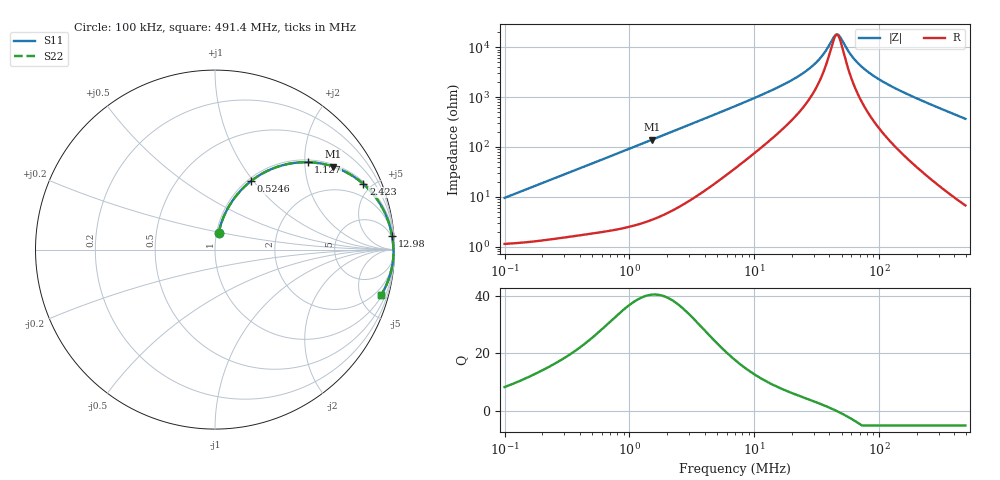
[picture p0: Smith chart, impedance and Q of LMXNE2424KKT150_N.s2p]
! LMXNE2424KKT150_N  S-PARAMETER MODEL  ( General Type )
! Model Generated by TAIYO YUDEN Corporation (http://www.ty-top.com)
! Version 1.0
! TAIYO YUDEN Control No. 191023NI43SB-FBB
! Copyright(c) 2019 TAIYO YUDEN CO.,LTD. All Rights Reserved.
! Product Description (link to TY-COMPAS)
! https://ds.yuden.co.jp/TYCOMPAS/or/detail?pn=LMXNE2424KKT150MN&u=M
! Products Name : Inductors
! Characteristics :
!  Inductance : 15 uH , SRF(min) : 27 MHz , DC Resistance(max) : 1.224 Ohm
!  Rated Current : Saturation :470 mA , Temp Rise : 370 mA
!  Case Size : 2.4 x 2.4 / 0.094 x 0.094 [mm/inch] , Thickness : 1 / 0.039 [mm/inch]
!  (Conditions: Temperature = 25 degC , DC Bias Current/Voltage = 0A / 0V)
! External Node Assignments :
!  1  o---GGG---o  2
! GND o---------o GND
! Frequency Range : 0.1MHz  -  491.415554MHz  [ 402 STEP ]
# MHz S RI R 50
! Freq[MHz].  S11 Real  S11 Imag  S21 Real  S21 Imag  S12 Real  S12 Imag  S22 Real  S22 Imag
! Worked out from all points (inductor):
!   401 points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, 100 kHz to 491.4 MHz, reference 50 ohm
!   read as one part in series: L = 15 uH near 104.3 kHz
!   highest Q = 40.4 at 1.518 MHz (marker M1), where L = 14.7 uH
!   self-resonance near 45.48 MHz
!   S11 on the Smith chart (normalised r, x): 100 kHz: 1.02, +0.19; 524.6 kHz: 1.04, +0.97; 1.127 MHz: 1.05, +2.08; 2.423 MHz: 1.12, +4.47; 12.98 MHz: 4, +25; 491.4 MHz: 1.13, -7.34
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0.1  0.0198 0.0916  0.9802 -0.0916  0.9802 -0.0916  0.0198 0.0916
0.229043  0.056 0.1998  0.944 -0.1998  0.944 -0.1998  0.056 0.1998
0.415258  0.1405 0.326  0.8595 -0.326  0.8595 -0.326  0.1405 0.326
0.524605  0.2003 0.3816  0.7997 -0.3816  0.7997 -0.3816  0.2003 0.3816
1.127361  0.5189 0.4868  0.4811 -0.4868  0.4811 -0.4868  0.5189 0.4868
1.517972  0.6582 0.4621  0.3418 -0.4621  0.3418 -0.4621  0.6582 0.4621
1.72439  0.7116 0.4408  0.2884 -0.4408  0.2884 -0.4408  0.7116 0.4408
2.422665  0.8266 0.3654  0.1734 -0.3654  0.1734 -0.3654  0.8266 0.3654
3.866545  0.9199 0.2546  0.0801 -0.2546  0.0801 -0.2546  0.9199 0.2546
7.010104  0.9695 0.1461  0.0305 -0.1461  0.0305 -0.1461  0.9695 0.1461
12.98239  0.9863 0.0763  0.0137 -0.0763  0.0137 -0.0763  0.9863 0.0763
21.16473  0.9913 0.0408  0.00871 -0.0408  0.00871 -0.0408  0.9913 0.0408
29.11  0.9931 0.0228  0.00692 -0.0228  0.00692 -0.0228  0.9931 0.0228
35.24518  0.9938 0.013  0.00617 -0.013  0.00617 -0.013  0.9938 0.013
43.58991  0.9944 0.0025  0.00559 -0.0025  0.00559 -0.0025  0.9944 0.0025
46.45921  0.9945 -0.000655  0.00547 0.000655  0.00547 0.000655  0.9945 -0.000655
49.51738  0.9946 -0.00382  0.00538 0.00382  0.00538 0.00382  0.9946 -0.00382
59.9536  0.9947 -0.0136  0.00525 0.0136  0.00525 0.0136  0.9947 -0.0136
69.56898  0.9947 -0.0215  0.00535 0.0215  0.00535 0.0215  0.9947 -0.0215
87.88818  0.9941 -0.0351  0.0059 0.0351  0.0059 0.0351  0.9941 -0.0351
120.8815  0.9923 -0.0569  0.00774 0.0569  0.00774 0.0569  0.9923 -0.0569
491.4156  0.927 -0.2512  0.073 0.2512  0.073 0.2512  0.927 -0.2512
